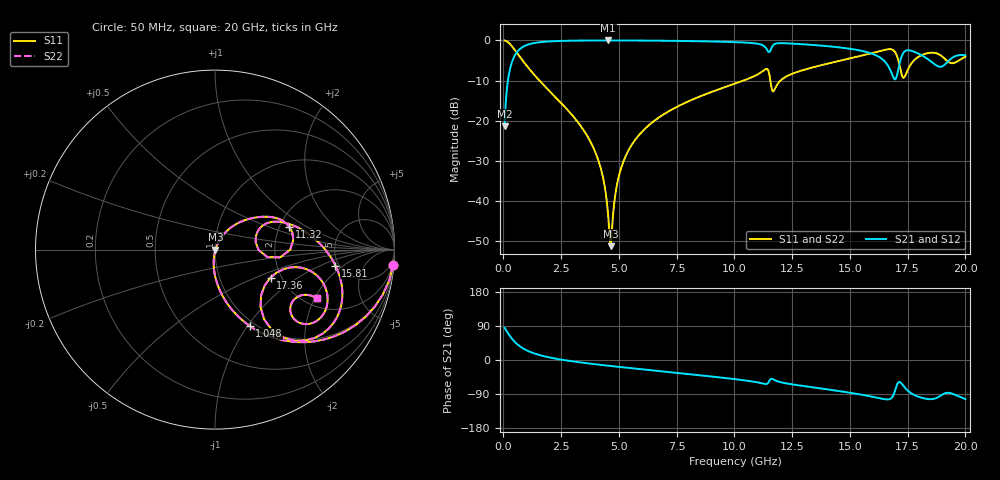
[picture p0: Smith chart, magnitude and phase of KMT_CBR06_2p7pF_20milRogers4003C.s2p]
! Data measured by Modelithics Inc. support@modelithics.com 813-866-6335
! KEMET CBR0603 2.7pF, Pad Width= 0.851mm, Pad Length= 0.64mm, Pad Gap= 0.62mm, 20mil Rogers 4003C substrate Data, January 2022
# hz S ma R 50
! 2 Port Network Data from SP1.SP block
! freq  magS11  angS11  magS21  angS21  magS12  angS12  magS22  angS22
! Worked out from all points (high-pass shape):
!   401 points, 50 MHz to 20 GHz, reference 50 ohm
!   highest |S21| = -0.03 dB at 4.539 GHz (marker M1); lowest = -21.3 dB at 50 MHz (marker M2)
!   |S21| within 3 dB of the highest: 573.5 MHz to 15.8 GHz (15.22 GHz wide, 186 % of centre); 17.33 GHz to 17.86 GHz (534 MHz wide, 3.03 % of centre)
!   lowest |S11| = -51.2 dB at 4.638 GHz (marker M3), VSWR 1.01, Z = 50.3 - j0.0706 ohm
!   |S11| at or under -10 dB: 1.558 GHz to 10.39 GHz (8.835 GHz wide, 148 % of centre); 11.55 GHz to 12 GHz (443.3 MHz wide, 3.76 % of centre)
!   |S22| runs from -51.2 to 0.0 dB; largest |S21 - S12| = 0
!   S11 on the Smith chart (normalised r, x): 50 MHz: 1, -22; 1.048 GHz: 0.94, -1.02; 11.32 GHz: 2.26, +0.71; 15.81 GHz: 4.66, -1.54; 17.36 GHz: 1.76, -0.62; 20 GHz: 2.31, -2.07
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5e7  0.9963 -5.1  0.08563 84.9  0.08563 84.9  0.9963 -5.1
2.495e8  0.9184 -24.1  0.3949 65.8  0.3949 65.8  0.9184 -24.1
3.99125e8  0.8224 -36.0  0.5681 54.0  0.5681 54.0  0.8224 -36.0
1.0475e9  0.467 -65.6  0.8829 24.3  0.8829 24.3  0.467 -65.6
3.391625e9  0.08239 -95.2  0.9942 -6.8  0.9942 -6.8  0.08239 -95.2
4.189625e9  0.02708 -97.2  0.9969 -12.7  0.9969 -12.7  0.02708 -97.2
4.53875e9  0.006375 -79.9  0.9971 -15.1  0.9971 -15.1  0.006375 -79.9
4.6385e9  0.002751 -14.8  0.9971 -15.8  0.9971 -15.8  0.002751 -14.8
4.93775e9  0.01722 62.7  0.9968 -17.8  0.9968 -17.8  0.01722 62.7
5.286875e9  0.03608 65.3  0.9962 -20.0  0.9962 -20.0  0.03608 65.3
6.73325e9  0.1099 59.1  0.9902 -29.1  0.9902 -29.1  0.1099 59.1
1.0025e10  0.2897 38.2  0.9506 -50.6  0.9506 -50.6  0.2897 38.2
1.132175e10  0.4335 17.0  0.8303 -63.2  0.8303 -63.2  0.4335 17.0
1.172075e10  0.2396 18.0  0.8931 -52.3  0.8931 -52.3  0.2396 18.0
1.336662e10  0.459 16.9  0.8778 -71.9  0.8778 -71.9  0.459 16.9
1.58105e10  0.6772 -7.6  0.704 -94.9  0.704 -94.9  0.6772 -7.6
1.670825e10  0.7772 -29.4  0.4505 -103.5  0.4505 -103.5  0.7772 -29.4
1.70075e10  0.6721 -49.0  0.3425 -70.0  0.3425 -70.0  0.6721 -49.0
1.735662e10  0.3464 -26.7  0.7224 -71.2  0.7224 -71.2  0.3464 -26.7
1.810475e10  0.6544 -19.4  0.6524 -99.7  0.6524 -99.7  0.6544 -19.4
1.890275e10  0.659 -39.1  0.4686 -95.1  0.4686 -95.1  0.659 -39.1
2e10  0.6278 -25.6  0.6537 -103.2  0.6537 -103.2  0.6278 -25.6
